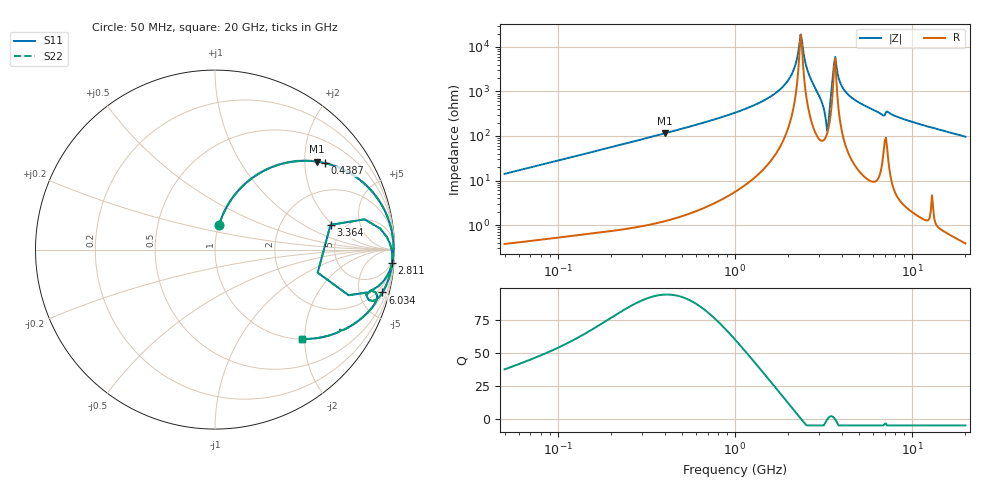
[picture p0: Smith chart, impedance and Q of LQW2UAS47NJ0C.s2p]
!Murata Part Number: LQW2UAS47NJ0C
!These Parameters are Measured in Series Mode Connection
!  o--[Z]--o
!Port1  Port2
!  o-------o
!Freq. Start=50[MHz] Stop=20[GHz], 401[Steps]
# Hz S RI R 50
!Freq.(Hz) S11(Real) S11(Imag) S21(Real) S21(Imag) S12(Real) S12(Imag) S22(Real) S22(Imag)
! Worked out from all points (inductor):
!   401 points, 50 MHz to 20 GHz, reference 50 ohm
!   read as one part in series: L = 44.7 nH near 51.52 MHz
!   highest Q = 94.1 at 401 MHz (marker M1), where L = 45.5 nH
!   self-resonance near 2.349 GHz
!   S11 on the Smith chart (normalised r, x): 50 MHz: 1.01, +0.28; 438.7 MHz: 1.03, +2.52; 2.811 GHz: 4, -26; 3.364 GHz: 3.88, +1.89; 6.034 GHz: 1.19, -7.77; 20 GHz: 1.01, -1.93
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5e7  0.023 0.1373  0.977 -0.1373  0.977 -0.1373  0.023 0.1373
1.364002e8  0.1314 0.33  0.8686 -0.33  0.8686 -0.33  0.1314 0.33
3.721004e8  0.5286 0.4939  0.4714 -0.4939  0.4714 -0.4939  0.5286 0.4939
4.010383e8  0.567 0.4902  0.433 -0.4902  0.433 -0.4902  0.567 0.4902
4.387496e8  0.6125 0.4819  0.3875 -0.4819  0.3875 -0.4819  0.6125 0.4819
1e9  0.9136 0.2727  0.0864 -0.2727  0.0864 -0.2727  0.9136 0.2727
1.476162e9  0.9725 0.1494  0.0275 -0.1494  0.0275 -0.1494  0.9725 0.1494
1.875929e9  0.9897 0.0747  0.0103 -0.0747  0.0103 -0.0747  0.9897 0.0747
2.114743e9  0.9939 0.0365  0.00611 -0.0365  0.00611 -0.0365  0.9939 0.0365
2.348516e9  0.9949 0.00106  0.0051 -0.00106  0.0051 -0.00106  0.9949 0.00106
2.728004e9  0.9895 -0.0598  0.0105 0.0598  0.0105 0.0598  0.9895 -0.0598
2.810964e9  0.9863 -0.0757  0.0137 0.0757  0.0137 0.0757  0.9863 -0.0757
3.075291e9  0.9553 -0.152  0.0447 0.152  0.0447 0.152  0.9553 -0.152
3.216634e9  0.8571 -0.2373  0.1429 0.2373  0.1429 0.2373  0.8571 -0.2373
3.364474e9  0.6436 0.1378  0.3564 -0.1378  0.3564 -0.1378  0.6436 0.1378
3.572216e9  0.9727 0.0383  0.0273 -0.0383  0.0273 -0.0383  0.9727 0.0383
3.680849e9  0.985 -0.00665  0.015 0.00665  0.015 0.00665  0.985 -0.00665
3.967106e9  0.9876 -0.0678  0.0124 0.0678  0.0124 0.0678  0.9876 -0.0678
4.275624e9  0.9825 -0.1062  0.0175 0.1062  0.0175 0.1062  0.9825 -0.1062
6.034176e9  0.9328 -0.2386  0.0672 0.2386  0.0672 0.2386  0.9328 -0.2386
7.442007e9  0.9026 -0.27  0.0974 0.27  0.0974 0.27  0.9026 -0.27
2e10  0.4829 -0.4977  0.5171 0.4977  0.5171 0.4977  0.4829 -0.4977
